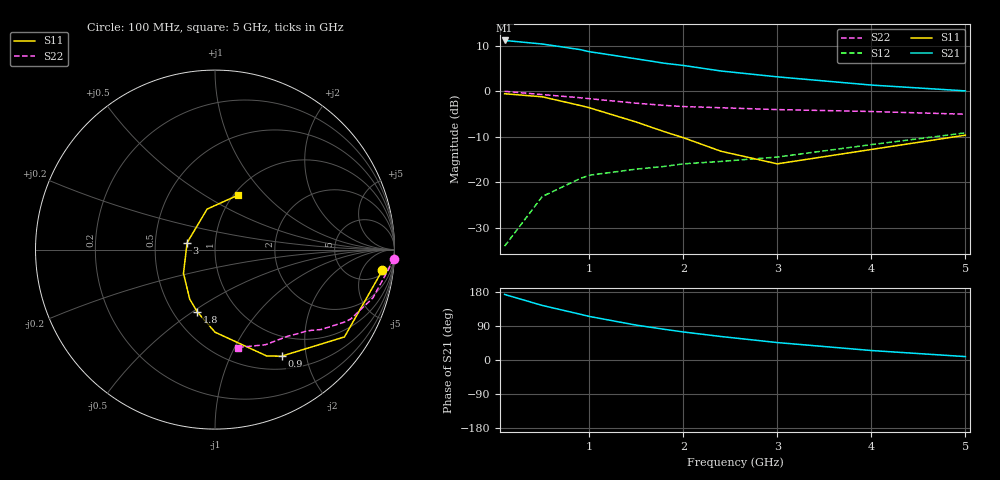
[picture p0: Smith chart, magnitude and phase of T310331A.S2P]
!AT-31033
!S and NOISE PARAMETERS at Vce=1V  Ic=1mA.  LAST UPDATED 06-23-94
# ghz s ma r 50
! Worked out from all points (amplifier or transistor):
!   11 points, 100 MHz to 5 GHz, reference 50 ohm
!   highest |S21| = 11.2 dB at 100 MHz (marker M1)
!   |S21| within 3 dB of that: start of sweep to 1.172 GHz
!   unconditionally stable (mu >= 1): 2.284 GHz to 4.327 GHz
!   at 500 MHz: K = 0.29, MSG = 16.7 dB, |S12| = -23.1 dB
!   at 1.8 GHz: K = 0.88, MSG = 11.3 dB, |S12| = -16.5 dB
!   at 5 GHz: K = 0.95, MSG = 4.6 dB, |S12| = -9.1 dB
!   lowest NFmin = 0.50 dB at 500 MHz
!   S11 on the Smith chart (normalised r, x): 100 MHz: 7, -13; 900 MHz: 0.68, -1.59; 1.8 GHz: 0.66, -0.52; 3 GHz: 0.73, +0.06; 5 GHz: 1.05, +0.71
0.1  0.94 -7.0  3.61 173.0  0.02 85.0  0.999 -3.0
0.5  0.87 -34.0  3.3 144.0  0.07 68.0  0.92 -17.0
0.9  0.7 -58.0  2.87 121.0  0.11 56.0  0.85 -27.0
1  0.66 -64.0  2.72 115.0  0.12 53.0  0.83 -29.0
1.5  0.46 -90.0  2.27 92.0  0.14 45.0  0.74 -37.0
1.8  0.36 -106.0  2.03 81.0  0.15 43.0  0.7 -40.0
2  0.31 -117.0  1.92 74.0  0.16 42.0  0.68 -42.0
2.4  0.22 -143.0  1.67 62.0  0.17 42.0  0.66 -45.0
3  0.16 166.0  1.44 46.0  0.19 44.0  0.63 -50.0
4  0.23 101.0  1.17 25.0  0.26 46.0  0.6 -62.0
5  0.33 67.0  1.01 9.0  0.35 41.0  0.56 -77.0
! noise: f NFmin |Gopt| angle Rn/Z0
0.5  0.5  0.9  12  0.7
0.9  0.6  0.82  28  0.6
1.8  1.1  0.57  68  0.38
2.4  1.6  0.41  100  0.22
